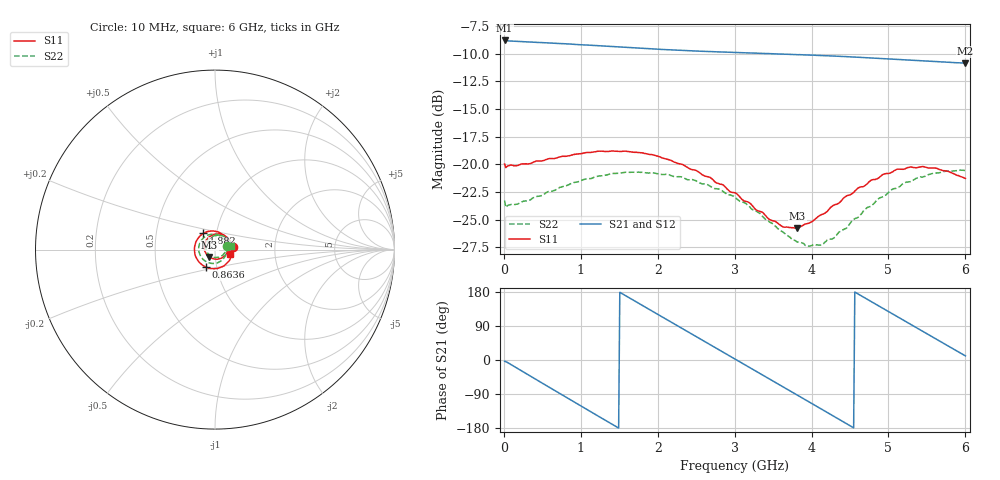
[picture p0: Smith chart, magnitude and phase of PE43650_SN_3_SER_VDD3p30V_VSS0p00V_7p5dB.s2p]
!Keysight Technologies,N5245B,MY57181451,A.13.50.07
!Date: Tuesday, May 07, 2019 07:59:59
!Correction: S11(Full 2 Port(1,2))
!S21(Full 2 Port(1,2))
!S12(Full 2 Port(1,2))
!S22(Full 2 Port(1,2))
!S2P File: Measurements: S11, S21, S12, S22:
# Hz S  dB  R 50
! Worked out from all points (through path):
!   401 points, 10 MHz to 6 GHz, reference 50 ohm
!   highest |S21| = -8.81 dB at 10 MHz (marker M1); lowest = -10.9 dB at 6 GHz (marker M2)
!   group delay of S21, straight-line fit = 327 ps
!   lowest |S11| = -25.8 dB at 3.814 GHz (marker M3), VSWR 1.11, Z = 46.8 - j3.84 ohm
!   |S11| at or under -10 dB: start of sweep to end of sweep
!   |S22| runs from -27.4 to -20.5 dB; largest |S21 - S12| = 0.003
!   S11 on the Smith chart (normalised r, x): 10 MHz: 1.22, +0.04; 863.6 MHz: 0.88, -0.17; 1.882 GHz: 0.87, +0.16; 6 GHz: 1.18, -0.06
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1e7  -19.98 8.8  -8.81 -3.4  -8.88 -3.3  -23.27 16.9
2.34625e8  -19.96 -34.4  -8.91 -29.1  -8.96 -29.1  -23.40 -33.8
4.892e8  -19.70 -69.7  -8.99 -59.9  -9.05 -59.8  -22.83 -69.3
8.63575e8  -19.20 -118.8  -9.13 -104.8  -9.19 -104.8  -21.77 -116.4
1.013325e9  -19.03 -137.2  -9.20 -122.6  -9.25 -122.7  -21.44 -133.6
1.4476e9  -18.81 172.8  -9.37 -174.2  -9.43 -174.2  -20.83 -179.4
1.881875e9  -19.09 125.5  -9.55 134.5  -9.61 134.5  -20.79 137.9
2.01665e9  -19.30 111.4  -9.60 118.6  -9.65 118.6  -20.87 125.3
2.241275e9  -19.87 87.4  -9.68 92.2  -9.74 92.3  -21.14 103.8
2.4659e9  -20.50 62.7  -9.75 65.9  -9.81 65.9  -21.42 82.4
2.750425e9  -21.62 31.5  -9.83 32.5  -9.88 32.6  -22.21 54.1
3.005e9  -22.58 -0.4  -9.89 2.7  -9.95 2.7  -22.97 27.5
3.45425e9  -25.00 -64.8  -10.00 -50.2  -10.04 -50.1  -25.22 -28.2
3.81365e9  -25.77 -127.4  -10.09 -92.5  -10.14 -92.4  -27.03 -82.9
4.008325e9  -25.18 -160.9  -10.13 -115.4  -10.18 -115.4  -27.33 -117.4
4.277875e9  -23.73 158.1  -10.21 -147.2  -10.27 -147.1  -26.71 -164.1
4.517475e9  -22.70 125.6  -10.29 -175.5  -10.35 -175.3  -25.18 158.2
4.757075e9  -21.53 96.8  -10.39 156.3  -10.44 156.5  -23.83 128.4
5.01165e9  -20.81 69.9  -10.48 126.5  -10.53 126.7  -22.45 98.7
5.4609e9  -20.22 26.9  -10.65 73.8  -10.70 74.0  -21.11 55.6
5.745425e9  -20.61 3.0  -10.77 40.5  -10.81 40.7  -20.63 31.1
6e9  -21.28 -15.8  -10.86 10.9  -10.91 10.9  -20.57 11.2
